(* Logix 5000 AddOnInstructionDefinition export AMCI_ANG1E_Absolute_Move; software revision 20.05 *)

ADD_ON_INSTRUCTION AMCI_ANG1E_Absolute_Move   (* revision 6.1, vendor AMCI, ExecuteEnableInFalse *)
// Revision note:
// Version 5.0 added the (hidden) ability to program the motor current and unlatched the error bit if the rung goes false.
// 8/5/2019.  Version 6 automatically issued the reset error command if the move complete bit was set.  This will reset the move complete bit and allow short moves to occur.
// 7/31/23 V6.1 Changed how the AOI EN bit is set.   Instead of when the Move complete bit is not set, it is now set when the move command is issued.
VAR_INPUT
   Axis_Status_Bits : INT; {required}
   slot_axis_number : INT; {required}
   Type_0_for_standard_1_for_indexed : BOOL;
   Target_Position : DINT; {required}
   Programmed_Speed : DINT; {required}
   Acceleration : INT; {required}
   Deceleration : INT; {required}
   motor_current : INT;
   Jerk : INT;
END_VAR
VAR_IN_OUT
   AMCI_ANG1E_output_data : INT[10]; {required}
END_VAR
VAR_OUTPUT
   EN : BOOL; {access Read Only, visible}
   ER : BOOL; {access Read Only, visible}
END_VAR
VAR
   Upper_Result_X_1000 : DINT;
   command_data_block : INT[10];
        [0]   // Command Bits MSW
        [1]   // Command Bits LSW
        [2]   // Upper Target Position
        [3]   // Lower Target Position
        [4]   // Upper Programmed Speed
        [5]   // Lower Programmed Speed
   index : INT;
END_VAR

ROUTINE EnableInFalse   (* ladder *)
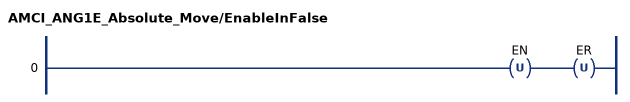
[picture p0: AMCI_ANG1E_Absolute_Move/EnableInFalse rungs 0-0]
   0: OTU(EN)OTU(ER);
END_ROUTINE

ROUTINE Logic   (* ladder *)
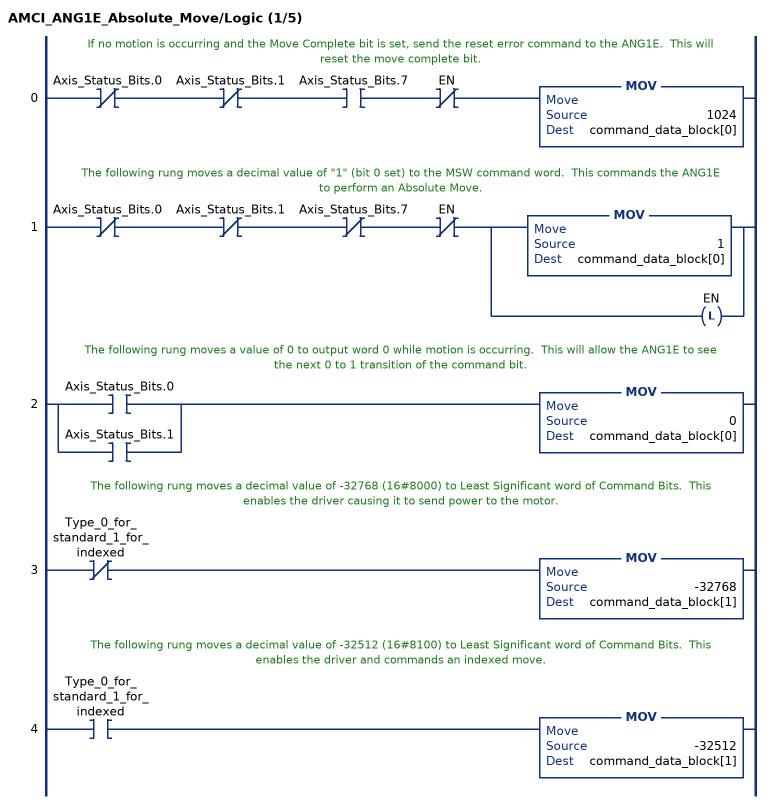
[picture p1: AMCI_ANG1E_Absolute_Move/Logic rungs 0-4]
   // If no motion is occurring and the Move Complete bit is set, send the reset error command to the ANG1E.  This will reset the move complete bit.
   0: XIO(Axis_Status_Bits.0)XIO(Axis_Status_Bits.1)XIC(Axis_Status_Bits.7)XIO(EN)MOV(1024,command_data_block[0]);
   // The following rung moves a decimal value of "1" (bit 0 set) to the MSW command word.  This commands the ANG1E to perform an Absolute Move.
   1: XIO(Axis_Status_Bits.0)XIO(Axis_Status_Bits.1)XIO(Axis_Status_Bits.7)XIO(EN)[MOV(1,command_data_block[0]) ,OTL(EN) ];
   // The following rung moves a value of 0 to output word 0 while motion is occurring.  This will allow the ANG1E to see the next 0 to 1 transition of the command bit.
   2: [XIC(Axis_Status_Bits.0) ,XIC(Axis_Status_Bits.1) ]MOV(0,command_data_block[0]);
   // The following rung moves a decimal value of -32768 (16#8000) to Least Significant word of Command Bits.  This enables the driver causing it to send power to the motor.
   3: XIO(Type_0_for_standard_1_for_indexed)MOV(-32768,command_data_block[1]);
   // The following rung moves a decimal value of -32512 (16#8100) to Least Significant word of Command Bits.  This enables the driver and commands an indexed move.
   4: XIC(Type_0_for_standard_1_for_indexed)MOV(-32512,command_data_block[1]);
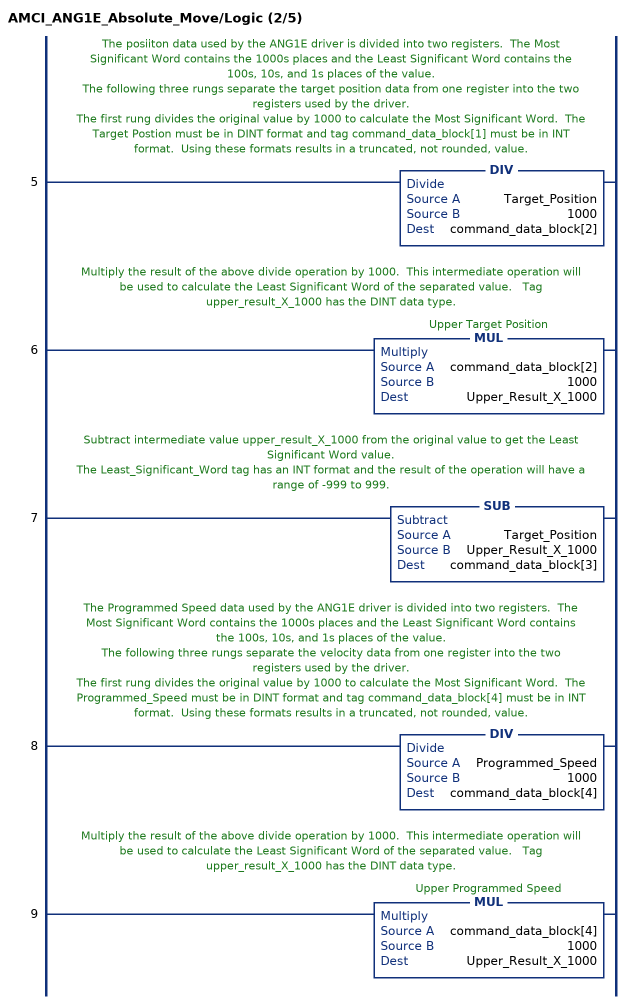
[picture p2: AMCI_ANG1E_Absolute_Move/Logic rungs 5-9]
   // The posiiton data used by the ANG1E driver is divided into two registers.  The Most Significant Word contains the 1000s places and the Least Significant Word contains the 100s, 10s, and 1s places of the value.
   // The following three rungs separate the target position data from one register into the two registers used by the driver.
   // The first rung divides the original value by 1000 to calculate the Most Significant Word.  The Target Postion must be in DINT format and tag command_data_block[1] must be in INT format.  Using these formats results in a truncated, not rounded, value.
   5: DIV(Target_Position,1000,command_data_block[2]);
   // Multiply the result of the above divide operation by 1000.  This intermediate operation will be used to calculate the Least Significant Word of the separated value.   Tag upper_result_X_1000 has the DINT data type.
   6: MUL(command_data_block[2],1000,Upper_Result_X_1000);
   // Subtract intermediate value upper_result_X_1000 from the original value to get the Least Significant Word value.
   // The Least_Significant_Word tag has an INT format and the result of the operation will have a range of -999 to 999.
   7: SUB(Target_Position,Upper_Result_X_1000,command_data_block[3]);
   // The Programmed Speed data used by the ANG1E driver is divided into two registers.  The Most Significant Word contains the 1000s places and the Least Significant Word contains the 100s, 10s, and 1s places of the value.
   // The following three rungs separate the velocity data from one register into the two registers used by the driver.
   // The first rung divides the original value by 1000 to calculate the Most Significant Word.  The Programmed_Speed must be in DINT format and tag command_data_block[4] must be in INT format.  Using these formats results in a truncated, not rounded, value.
   8: DIV(Programmed_Speed,1000,command_data_block[4]);
   // Multiply the result of the above divide operation by 1000.  This intermediate operation will be used to calculate the Least Significant Word of the separated value.   Tag upper_result_X_1000 has the DINT data type.
   9: MUL(command_data_block[4],1000,Upper_Result_X_1000);
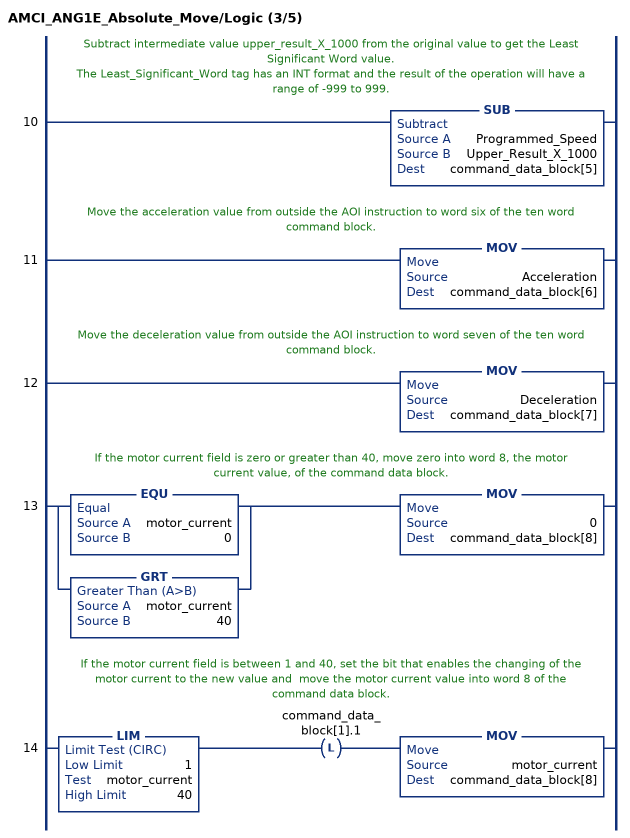
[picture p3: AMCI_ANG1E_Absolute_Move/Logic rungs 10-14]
   // Subtract intermediate value upper_result_X_1000 from the original value to get the Least Significant Word value.
   // The Least_Significant_Word tag has an INT format and the result of the operation will have a range of -999 to 999.
   10: SUB(Programmed_Speed,Upper_Result_X_1000,command_data_block[5]);
   // Move the acceleration value from outside the AOI instruction to word six of the ten word command block.
   11: MOV(Acceleration,command_data_block[6]);
   // Move the deceleration value from outside the AOI instruction to word seven of the ten word command block.
   12: MOV(Deceleration,command_data_block[7]);
   // If the motor current field is zero or greater than 40, move zero into word 8, the motor current value, of the command data block.
   13: [EQU(motor_current,0) ,GRT(motor_current,40) ]MOV(0,command_data_block[8]);
   // If the motor current field is between 1 and 40, set the bit that enables the changing of the motor current to the new value and  move the motor current value into word 8 of the command data block.
   14: LIM(1,motor_current,40)OTL(command_data_block[1].1)MOV(motor_current,command_data_block[8]);
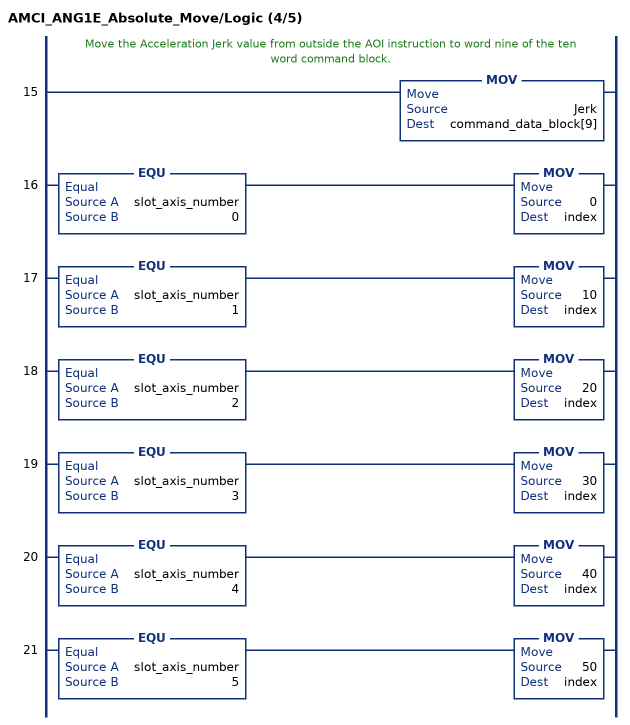
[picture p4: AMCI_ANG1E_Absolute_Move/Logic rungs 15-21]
   // Move the Acceleration Jerk value from outside the AOI instruction to word nine of the ten word command block.
   15: MOV(Jerk,command_data_block[9]);
   16: EQU(slot_axis_number,0)MOV(0,index);
   17: EQU(slot_axis_number,1)MOV(10,index);
   18: EQU(slot_axis_number,2)MOV(20,index);
   19: EQU(slot_axis_number,3)MOV(30,index);
   20: EQU(slot_axis_number,4)MOV(40,index);
   21: EQU(slot_axis_number,5)MOV(50,index);
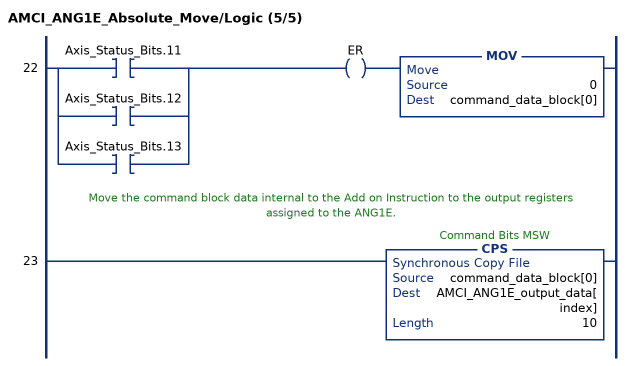
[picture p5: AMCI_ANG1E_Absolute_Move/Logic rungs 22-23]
   22: [XIC(Axis_Status_Bits.11) ,XIC(Axis_Status_Bits.12) ,XIC(Axis_Status_Bits.13) ]OTE(ER)MOV(0,command_data_block[0]);
   // Move the command block data internal to the Add on Instruction to the output registers assigned to the ANG1E.
   23: CPS(command_data_block[0],AMCI_ANG1E_output_data[index],10);
END_ROUTINE
END_ADD_ON_INSTRUCTION
